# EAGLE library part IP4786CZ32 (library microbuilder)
IP4786CZ32
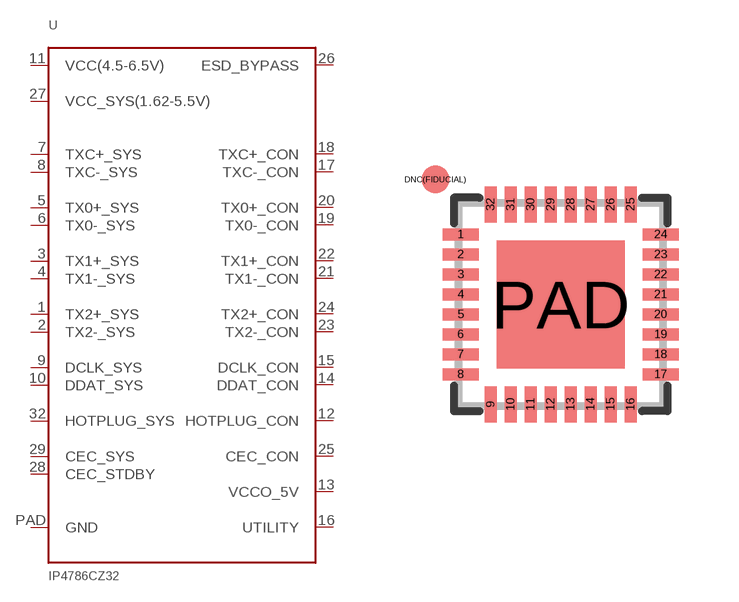
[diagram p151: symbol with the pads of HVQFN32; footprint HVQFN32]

Designator prefix U

## IP4786CZ32  [HVQFN32]
1  TX2+_SYS
2  TX2-_SYS
3  TX1+_SYS
4  TX1-_SYS
5  TX0+_SYS
6  TX0-_SYS
7  TXC+_SYS
8  TXC-_SYS
9  DCLK_SYS
10  DDAT_SYS
11  VCC(4.5-6.5V)
12  HOTPLUG_CON
13  VCCO_5V
14  DDAT_CON
15  DCLK_CON
16  UTILITY
17  TXC-_CON
18  TXC+_CON
19  TX0-_CON
20  TX0+_CON
21  TX1-_CON
22  TX1+_CON
23  TX2-_CON
24  TX2+_CON
25  CEC_CON
26  ESD_BYPASS
27  VCC_SYS(1.62-5.5V)
28  CEC_STDBY
29  CEC_SYS
32  HOTPLUG_SYS
PAD  GND

## Footprint HVQFN32 (pad centres in mm)
HVQFN32 SOT617-1 JEDEC MO-220
smd 0.9 x 0.3: 1 -2.5,1.75; 2 -2.5,1.25; 3 -2.5,0.75; 4 -2.5,0.25; 5 -2.5,-0.25; 6 -2.5,-0.75; 7 -2.5,-1.25; 8 -2.5,-1.75; 17 2.5,-1.75; 18 2.5,-1.25; 19 2.5,-0.75; 20 2.5,-0.25; 21 2.5,0.25; 22 2.5,0.75; 23 2.5,1.25; 24 2.5,1.75
smd 0.3 x 0.9: 9 -1.75,-2.5; 10 -1.25,-2.5; 11 -0.75,-2.5; 12 -0.25,-2.5; 13 0.25,-2.5; 14 0.75,-2.5; 15 1.25,-2.5; 16 1.75,-2.5; 25 1.75,2.5; 26 1.25,2.5; 27 0.75,2.5; 28 0.25,2.5; 29 -0.25,2.5; 30 -0.75,2.5; 31 -1.25,2.5; 32 -1.75,2.5
smd 0.7 x 0.7: DNC(FIDUCIAL) -3.127,3.127
smd 3.2 x 3.2: PAD 0,0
